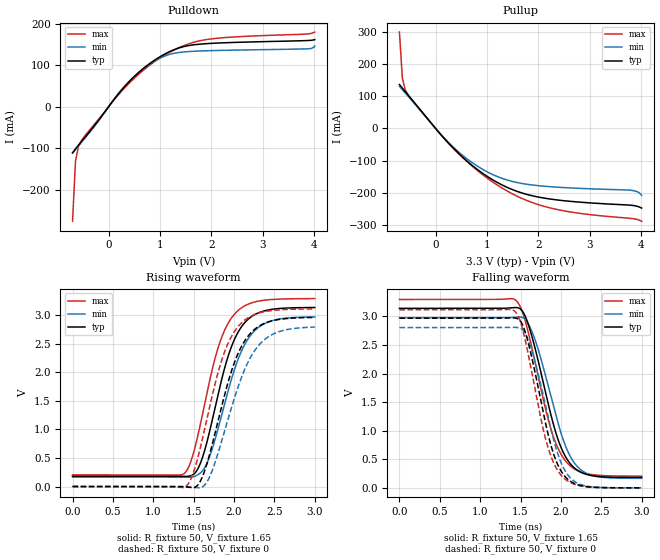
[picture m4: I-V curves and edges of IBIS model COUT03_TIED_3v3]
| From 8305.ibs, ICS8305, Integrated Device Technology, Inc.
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[Model] COUT03_TIED_3v3
Model_type   Output
Polarity   Non-Inverting
|   typ   min   max
C_comp   2pF   1.5pF   2.5pF
Vmeas = 1.65V
Rref = 50
Cref = 0
Vref = 1.65V
|   typ   min   max
[Voltage range]   3.3V   3.135V   3.465V
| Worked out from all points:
|   slope of the pulldown table from 0 to 0.495 V, typ, clamps not added: 6.88 ohm
|   slope of the pullup table from 0 to 0.495 V, typ, clamps not added: 5.83 ohm
|   rising waveform, R_fixture 50, V_fixture 1.65: 20-80 % time 332ps typ, 360ps min, 324ps max; typ from 0.181 V to 3.14 V
|   falling waveform, R_fixture 50, V_fixture 1.65: 20-80 % time 322ps typ, 338ps min, 322ps max; typ from 3.14 V to 0.181 V
|   rising waveform, R_fixture 50, V_fixture 0: 20-80 % time 359ps typ, 397ps min, 347ps max; typ from 0 V to 2.96 V
|   falling waveform, R_fixture 50, V_fixture 0: 20-80 % time 285ps typ, 297ps min, 286ps max; typ from 2.97 V to 0 V
[Pulldown]
|Voltage   I (typ)   I (min)   I (max)
|Note, modeling breaks down at 250mA and above.  This is well beyond the functional   |
|operating range of the device.  Should this scenario occur, catastrophic failure and   |
|possible damage to the device and/or board is of higher concern than the I-V curve   |
|behavior.  The IBIS checker will flag currents in excess of 10A with warnings.  Lines   |
|with currents in excess of 0.35 A have been commented out.  The points still remain|
|available to the user if the user desires to use them.   |
|-2.84000e+00   -2.38215e+01   -2.89470e+01   -1.92821e+01
|-2.38000e+00   -1.83770e+01   -2.20062e+01   -1.51871e+01
|-1.92000e+00   -1.29278e+01   -1.50613e+01   -1.10891e+01
|-1.46000e+00   -7.47412e+00   -8.10966e+00   -6.98753e+00
|-1.00000e+00   -2.01652e+00   -1.15380e+00   -2.88245e+00
|-9.90000e-01   -1.89785e+00   -1.00258e+00   -2.79318e+00
|-9.32644e-01   -1.21724e+00   -2.53878e-01   -2.28116e+00
|-8.75287e-01   -5.36673e-01   -1.44386e-01   -1.76914e+00
|-8.17931e-01   -1.75032e-01   -1.29205e-01   -1.25713e+00
|-7.60575e-01   -1.25660e-01   -1.19756e-01   -7.45167e-01
-703.2mV  -111.8mA   -111mA     -276.2mA
-645.9mV  -102mA     -102.7mA   -130.9mA
-588.5mV  -92.88mA   -94.41mA   -95.88mA
-473.8mV  -75.61mA   -77.66mA   -71.94mA
271.8mV   42.81mA    43.92mA    39.92mA
730.7mV   97.37mA    96.68mA    93.3mA
1.19V     132.6mA    126mA      131.1mA
1.476V    145.1mA    131.8mA    147.5mA
1.763V    150.3mA    133.9mA    158.3mA
2.394V    154.4mA    136mA      167.4mA
3.885V    159.3mA    139.4mA    175.3mA
4.01V     161.4mA    146.3mA    179.6mA
| 4.52800e+00   6.95659e+00   1.05624e+01   5.05397e+00
| 5.04600e+00   1.63587e+01   2.25722e+01   1.21055e+01
| 5.56400e+00   2.57852e+01   3.46127e+01   1.91748e+01
| 6.08200e+00   3.52550e+01   4.67072e+01   2.62737e+01
| 6.60000e+00   4.48073e+01   5.88986e+01   3.34313e+01
[Pullup]
|Voltage   I (typ)   I (min)   I (max)
|Note, modeling breaks down at 250mA and above.  This is well beyond the functional   |
|operating range of the device.  Should this scenario occur, catastrophic failure and   |
|possible damage to the device and/or board is of higher concern than the I-V curve   |
|behavior.  The IBIS checker will flag currents in excess of 10A with warnings.  Lines   |
|with currents in excess of 0.35 A have been commented out.  The points still remain|
|available to the user if the user desires to use them.   |
|-2.84000e+00   3.63590e+01   4.42554e+01   2.93861e+01
|-2.38000e+00   2.79852e+01   3.35749e+01   2.30878e+01
|-1.92000e+00   1.96083e+01   2.28907e+01   1.67884e+01
|-1.46000e+00   1.12279e+01   1.22021e+01   1.04875e+01
|-1.00000e+00   2.84387e+00   1.50900e+00   4.18491e+00
|-9.90000e-01   2.66157e+00   1.27650e+00   4.04787e+00
|-9.32644e-01   1.61593e+00   2.75982e-01   3.26189e+00
|-8.75287e-01   5.74198e-01   1.67725e-01   2.47589e+00
|-8.17931e-01   2.01302e-01   1.51836e-01   1.68987e+00
|-7.60575e-01   1.51618e-01   1.41205e-01   9.03829e-01
-703.2mV  136.6mA    130.8mA    299.8mA
-645.9mV  125.2mA    120.4mA    155.5mA
-588.5mV  114.2mA    109.9mA    119.4mA
-531.1mV  103.2mA    99.34mA    103.6mA
271.8mV   -49.4mA    -46.9mA    -49.24mA
902.8mV   -138.2mA   -126.1mA   -142.3mA
1.476V    -189.1mA   -164.2mA   -201.9mA
2.05V     -215mA     -178.8mA   -239.5mA
2.738V    -228.4mA   -185.9mA   -262.6mA
3.771V    -238.5mA   -191.9mA   -279.5mA
3.943V    -243.2mA   -198mA     -284mA
4.01V     -247.8mA   -208.6mA   -288.8mA
| 4.52800e+00   -4.81923e+00   -7.12749e+00   -3.61019e+00
| 5.04600e+00   -1.09389e+01   -1.49354e+01   -8.20734e+00
| 5.56400e+00   -1.70599e+01   -2.27441e+01   -1.28068e+01
| 6.08200e+00   -2.31807e+01   -3.05527e+01   -1.74063e+01
| 6.60000e+00   -2.93014e+01   -3.83616e+01   -2.20056e+01
[Ramp]
|   typ   min   max
dV/dt_r   1.777/0.332n   1.686/0.36n   1.857/0.323n
dV/dt_f   1.784/0.323n   1.693/0.339n   1.864/0.323n
R_load =   50.0000
[Rising Waveform]
R_fixture = 50
V_fixture = 1.65   |Vcc_typ
V_fixture_min = 1.5675 |Vcc_min
V_fixture_max = 1.7325 |Vcc_max
C_fixture = 0.0p
| Time   typ   min   max
0s        180.7mV    165.9mV    204mV
1.348ns   179.6mV    166.2mV    206.1mV
1.496ns   209.9mV    168.7mV    576mV
1.586ns   415.6mV    239.9mV    1.106V
1.688ns   909mV      487mV      1.79V
1.829ns   1.772V     1.156V     2.546V
1.985ns   2.514V     1.962V     2.987V
2.138ns   2.882V     2.504V     3.173V
2.318ns   3.055V     2.806V     3.255V
3ns       3.139V     2.974V     3.295V
[Falling Waveform]
R_fixture = 50
V_fixture = 1.65   |Vcc_typ
V_fixture_min = 1.5675 |Vcc_min
V_fixture_max = 1.7325 |Vcc_max
C_fixture = 0.0p
| Time   typ   min   max
0s        3.141V     2.977V     3.296V
1.435ns   3.155V     2.987V     3.289V
1.544ns   3.046V     2.966V     2.992V
1.655ns   2.581V     2.69V      2.366V
1.868ns   1.324V     1.645V     1.068V
1.955ns   885.7mV    1.181V     721mV
2.042ns   583.9mV    788.4mV    499.4mV
2.168ns   346.1mV    433.1mV    329.4mV
2.321ns   233.3mV    250.9mV    246.9mV
3ns       181mV      166.3mV    204.3mV
[Rising Waveform]
R_fixture = 50
V_fixture =   0
V_fixture_min = 0
V_fixture_max = 0
C_fixture = 0.0p
| Time   typ   min   max
0s        8.011nV    6.832nV    6.445uV
1.375ns   -3.947mV   241.2uV    -16.71mV
1.529ns   -4.261mV   -19.16mV   386.7mV
1.613ns   185.8mV    -3.514mV   859mV
1.709ns   621.7mV    205.5mV    1.464V
1.868ns   1.522V     898.9mV    2.302V
2.033ns   2.277V     1.675V     2.774V
2.198ns   2.678V     2.249V     2.979V
2.381ns   2.864V     2.581V     3.067V
3ns       2.965V     2.796V     3.114V
[Falling Waveform]
R_fixture = 50
V_fixture =   0
V_fixture_min = 0
V_fixture_max = 0
C_fixture = 0.0p
| Time   typ   min   max
0s        2.968V     2.804V     3.115V
1.42ns    2.973V     2.809V     3.098V
1.52ns    2.869V     2.773V     2.808V
1.613ns   2.442V     2.517V     2.219V
1.811ns   1.124V     1.437V     852.9mV
1.895ns   657.1mV    924.9mV    486.9mV
1.979ns   353.2mV    524mV      264.6mV
2.093ns   140.7mV    212.2mV    110.9mV
2.243ns   39.45mV    57.58mV    34.21mV
3ns       58.51uV    63.95uV    92.67uV
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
